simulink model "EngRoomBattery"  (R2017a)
settings: Solver=VariableStepAuto  StartTime=0.0  StopTime=10.0  RelTol=1e-3
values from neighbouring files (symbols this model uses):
  EngDat = engine_pre()    [run_master.m]    (also in engine_pre.m = [MCR1, BSFC1, x)
undefined symbols (not defined in the file or in its folder): num

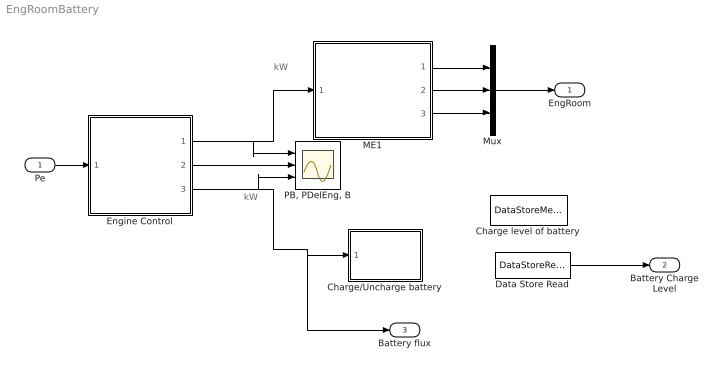
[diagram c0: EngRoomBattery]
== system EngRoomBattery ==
  note: kW
  note: kW
  Pe : Inport
  Charge level of battery : DataStoreMemory  DataStoreName=BatteryCharge  ReadBeforeWriteMsg=warning  WriteAfterWriteMsg=warning  WriteAfterReadMsg=warning  InitialValue=10000  ShowAdditionalParam=off  OutDataTypeStr=double
  Charge/Uncharge battery : MATLAB Function  TreatAsAtomicUnit=on
  Data Store Read : DataStoreRead  DataStoreName=BatteryCharge
  Engine Control : MATLAB Function  TreatAsAtomicUnit=on
  ME1 : MATLAB Function  TreatAsAtomicUnit=on
  Mux : Mux  Inputs=3
  "PB, PDelEng, B" : Scope  NumInputPorts=3
  EngRoom : Outport
  Battery Charge Level : Outport  Port=2
  Battery flux : Outport  Port=3
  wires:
  Pe/1 -> Engine Control/1(Pe)
  Engine Control/1(P1) -> "PB, PDelEng, B"/1, ME1/1("Pb ")
  ME1/1(fuel_cons) -> Mux/1
  ME1/3(x) -> Mux/3
  ME1/2(Pb) -> Mux/2
  Engine Control/3(B) -> "PB, PDelEng, B"/3, Battery flux/1, Charge/Uncharge battery/1(B)
  Data Store Read/1 -> Battery Charge Level/1
  Mux/1 -> EngRoom/1
  Engine Control/2(PdelEng) -> "PB, PDelEng, B"/2

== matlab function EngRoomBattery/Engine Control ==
function [P1, PdelEng, B]  = fcn(Pe,EngDat)
%take in the total propulsive powering need, and the optimal loading of the
%engine. Charge the battery if the demand is lower than MCR, and use the
%battery if the powering requirement is higher than MCR

Pe=Pe/1000; %Convert from W to kW
%capacity of each engine
PMCR1=EngDat(1,1);
xopt=EngDat(1,3);
%% Convert Pe into Pb required from the machinery
%eta_D = 0.55;
%eta_M = 0.95*0.98;
eta_T = 0.7;%eta_D* eta_M;   %Total efficiency
Pb = (Pe/eta_T); %kW required break power

PdelEng=xopt*PMCR1; %Power from engine at optimal load

if Pb>=PdelEng %Required power is higher than what engine produces
    diff=Pb-PdelEng; %Find the difference
    B=-diff; % power needed from battery [kW]
else
    diff=PdelEng-Pb; %surplus power generated from engine
    B=diff; % power going into battery
end
   
P1=Pb;
   
   
end

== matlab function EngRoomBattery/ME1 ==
function [fuel_cons, Pb, x] = fcn(Pb, num, EngDat)
%take in break power need [W], output fuel consumption [kg/h], Pb [W], and
%loading degree x [%]
PMCR=EngDat(1,1);
x = Pb/PMCR; %percentage of maximum
BSFC=EngDat(1,2); %g/kWh
delta_BSFC = 0;%6610.6*x^6 - 20524*x^5 + 23791*x^4 - 11985*x^3 + 1803.2*x^2 + 340.12*x - 36.733;


Pb=Pb*1; % [kW] 

Pb_cons=EngDat(1,1)*EngDat(1,3); %Engine Base Load
fuel_cons = ((delta_BSFC+BSFC)*(Pb_cons))/(1000); %[kg/hour]


end

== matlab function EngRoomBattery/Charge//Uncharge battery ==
function fcn(B)
batterycapacity=10000; %[kWh] - 10 MWh
global BatteryCharge

BatteryCharge = BatteryCharge + B;

if BatteryCharge >=batterycapacity %Battery can not go over capacity
    BatteryCharge=batterycapacity;
elseif BatteryCharge<=0
    BatteryCharge=0; %Battery can not go below zero charge
end
    
end
